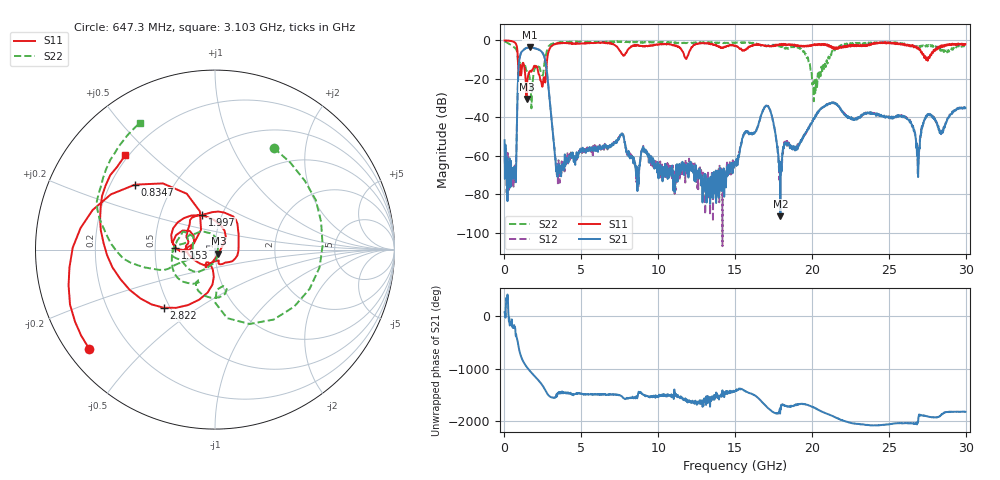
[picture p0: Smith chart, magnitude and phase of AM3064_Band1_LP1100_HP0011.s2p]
# Hz S DB R 50.0
!freq dBS11 angS11 dBS21 angS21 dBS12 angS12 dBS22 angS22
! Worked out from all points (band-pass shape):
!   1600 points, 10 MHz to 29.98 GHz, reference 50 ohm
!   highest |S21| = -3.68 dB at 1.678 GHz (marker M1); lowest = -91.3 dB at 17.95 GHz (marker M2)
!   |S21| within 3 dB of the highest: 1.067 GHz to 2.494 GHz (1.426 GHz wide, 80.1 % of centre)
!   lowest |S11| = -30.4 dB at 1.435 GHz (marker M3), VSWR 1.06, Z = 51.9 - j2.42 ohm
!   |S11| at or under -10 dB: 876.6 MHz to 2.775 GHz (1.898 GHz wide, 104 % of centre); 27.41528 GHz to 27.43728 GHz (22.01 MHz wide, 0.0802 % of centre); 27.51254 GHz to 27.55229 GHz (39.74 MHz wide, 0.144 % of centre)
!   |S22| runs from -35.3 to -0.5 dB; largest |S21 - S12| = 0.0087
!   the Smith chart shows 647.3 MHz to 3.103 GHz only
!   S11 on the Smith chart (normalised r, x): 647.3 MHz: 0.06, -0.35; 834.7 MHz: 0.30, +0.33; 1.153 GHz: 0.64, +0.01; 1.997 GHz: 0.81, +0.33; 2.822 GHz: 0.46, -0.37; 3.103 GHz: 0.19, +0.42
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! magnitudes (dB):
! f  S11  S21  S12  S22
! 10 MHz  -0.1  -51.9  -60.3  -0.5
! 647.3 MHz  -1.0  -68.6  -72.5  -3.7
! 834.7 MHz  -4.8  -34.1  -34.1  -6.8
! 1.153 GHz  -13.1  -5.6  -5.5  -12.9
! 1.435 GHz  -30.4  -4.0  -3.9  -15.9
! 1.678 GHz  -15.9  -3.7  -3.7  -21.9
! 1.997 GHz  -13.7  -4.2  -4.1  -14.3
! 2.822 GHz  -7.3  -21.0  -20.8  -3.9
! 3.103 GHz  -2.8  -43.9  -44.3  -1.7
! 3.553 GHz  -1.5  -68.9  -68.6  -1.1
! 5.015 GHz  -1.5  -57.3  -56.9  -0.6
! 7.639 GHz  -7.1  -48.9  -48.2  -0.7
! 8.613 GHz  -2.7  -66.8  -69.2  -0.9
! 10 GHz  -2.1  -67.5  -66.0  -1.0
! 15 GHz  -2.8  -64.0  -63.6  -1.4
! 17.05 GHz  -2.9  -33.9  -33.8  -3.0
! 17.95 GHz  -2.3  -91.3  -68.5  -2.8
! 19.99 GHz  -2.8  -43.0  -42.8  -18.2
! 25 GHz  -1.0  -40.1  -39.8  -1.2
! 26.89 GHz  -3.8  -68.5  -69.3  -3.4
! 27.49 GHz  -9.2  -39.5  -39.0  -2.9
! 29.98 GHz  -1.9  -35.0  -35.3  -3.0
